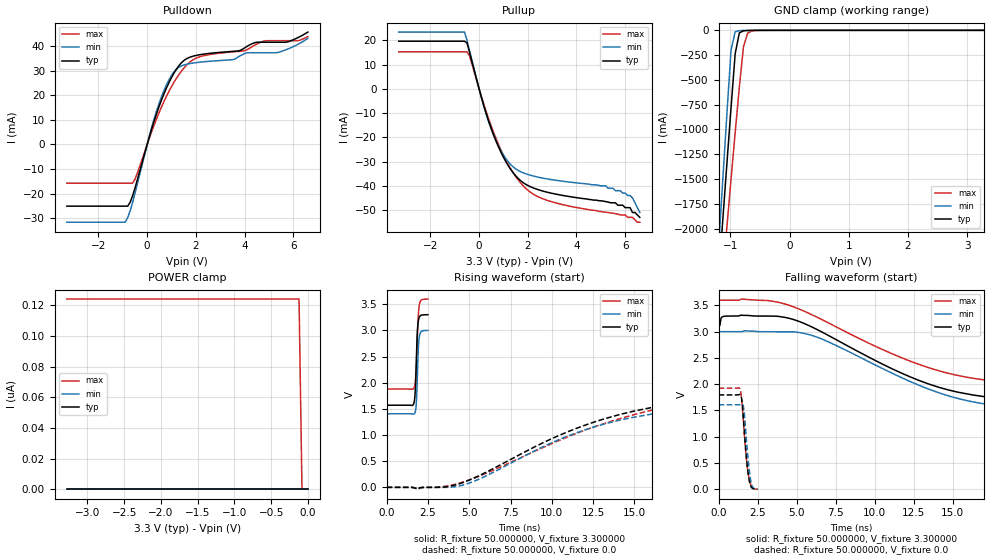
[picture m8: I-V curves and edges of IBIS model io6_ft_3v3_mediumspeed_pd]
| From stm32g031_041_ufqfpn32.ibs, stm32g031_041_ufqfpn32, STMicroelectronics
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|   Model io6_ft_3v3_mediumspeed_pd
[Model]  io6_ft_3v3_mediumspeed_pd
Model_type I/O
Polarity   Non-Inverting
Enable   Active-Low
Vinl =   0.990000V
Vinh =   2.310000V
Vmeas =  1.650000V
Cref =   50.000000pF
Rref =   100.000000M
Vref =   0.0V
C_comp   1.290400pF   1.272500pF   1.305600pF
[Temperature Range]   25.000000   -40.000000   0.125000k
[Pullup Reference]   3.300000V   3.000000V   3.600000V
[Pulldown Reference]   0.0V   0.0V   0.0V
[POWER Clamp Reference]   3.300000V   3.000000V   3.600000V
[GND Clamp Reference]   0.0V   0.0V   0.0V
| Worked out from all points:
|   slope of the pulldown table from 0 to 0.495 V, typ, clamps not added: 31.8 ohm
|   slope of the pullup table from 0 to 0.495 V, typ, clamps not added: 30.4 ohm
|   GND clamp passes 1 mA (typ) near -0.65 V on its own axis
|   rising waveform, R_fixture 50.000000, V_fixture 3.300000: 20-80 % time 114ps typ, 109ps min, 129ps max; typ from 1.57 V to 3.3 V
|   rising waveform, R_fixture 50.000000, V_fixture 0.0: 20-80 % time 8.23ns typ, 7.46ns min, 10.1ns max; typ from 0 V to 1.79 V
|   falling waveform, R_fixture 50.000000, V_fixture 3.300000: 20-80 % time 7.53ns typ, 7.46ns min, 8.06ns max; typ from 3.3 V to 1.57 V
|   falling waveform, R_fixture 50.000000, V_fixture 0.0: 20-80 % time 299ps typ, 288ps min, 331ps max; typ from 1.79 V to 0 V
[Pulldown]
|Voltage   I(typ)   I(min)   I(max)
-3.3V     -25.03mA   -31.54mA   -15.7mA
-900mV    -25.03mA   -31.54mA   -15.7mA
-700mV    -23.48mA   -26.95mA   -15.7mA
-500mV    -17.69mA   -19.75mA   -14.07mA
100mV     3.479mA    3.853mA    2.862mA
500mV     15.71mA    16.96mA    13.17mA
900mV     25.22mA    26.33mA    21.66mA
1.3V      31.91mA    31.32mA    28.29mA
2.2V      36.48mA    33.43mA    35.69mA
4.1V      39.78mA    37.21mA    38.43mA
5.4V      41.49mA    37.39mA    42.11mA
6.6V      45.6mA     43.05mA    43.74mA
[Pullup]
|Voltage   I(typ)   I(min)   I(max)
-3.3V     19.64mA    23.39mA    15.25mA
-600mV    19.64mA    23.39mA    15.25mA
-500mV    18.98mA    20.19mA    15.25mA
-400mV    15.37mA    16.06mA    13.73mA
100mV     -3.672mA   -3.825mA   -3.371mA
600mV     -19.12mA   -19.15mA   -18.08mA
1.2V      -31.74mA   -30.12mA   -31.25mA
1.8V      -38.62mA   -34.59mA   -39.86mA
3V        -43.11mA   -37.48mA   -46.63mA
5.8V      -48mA      -42mA      -52mA
6.3V      -51mA      -45mA      -53mA
6.6V      -53mA      -51mA      -55mA
[GND_clamp]
|Voltage   I(typ)   I(min)   I(max)
-3.3V     -9.61A     -9.635A    -9.699A
-1.2V     -2.493A    -2.184A    -2.958A
-1.13V    -1.917A    -1.512A    -2.469A
-1.06V    -1.345A    -845.6mA   -1.983A
-990mV    -779.8mA   -200.2mA   -1.503A
-920mV    -235.6mA   -14.2mA    -1.03A
-850mV    -26.08mA   -3.351mA   -574.2mA
-780mV    -4.512mA   -1.821mA   -166.4mA
-710mV    -1.735mA   -881.8uA   -29.46mA
-640mV    -819.4uA   -295.6uA   -6.294mA
3.28V     86.85uA    64.2uA     109.1uA
[POWER_clamp]
|Voltage   I(typ)   I(min)   I(max)
-3.28V    0A         0A         124nA
-120mV    0A         0A         124nA
-80mV     0A         0A         0A
0V        0A         0A         0A
[Ramp]
| variable   typ   min   max
dV/dt_r  1.07520/8.22726n   0.96294/7.44895n   1.14666/10.09657n
dV/dt_f  1.03122/14.35073n   0.95388/7.44449n   1.02582/8.04918n
R_load = 50.000000
[Rising Waveform]
R_fixture= 50.000000
V_fixture= 3.300000
V_fixture_min= 3.000000
V_fixture_max= 3.600000
|time   V(typ)   V(min)   V(max)
0s        1.57V      1.405V     1.878V
1.542ns   1.566V     1.403V     1.875V
1.657ns   1.62V      1.402V     1.904V
1.727ns   1.831V     1.438V     1.997V
1.792ns   2.386V     1.595V     2.294V
1.852ns   2.937V     2.054V     2.801V
1.917ns   3.182V     2.646V     3.293V
1.967ns   3.246V     2.852V     3.467V
2.052ns   3.283V     2.962V     3.562V
2.492ns   3.299V     2.999V     3.598V
[Rising Waveform]
R_fixture= 50.000000
V_fixture= 0.0
V_fixture_min= 0.0
V_fixture_max= 0.0
|time   V(typ)   V(min)   V(max)
0s        3.211nV    2.528nV    185.4nV
1.922ns   -21.16mV   -33.8mV    -31.31mV
3.604ns   10.6mV     -175.7uV   23.36mV
4.565ns   85.93mV    39.17mV    95.98mV
11.53ns   1.132V     1.047V     1.035V
14.25ns   1.403V     1.294V     1.324V
16.74ns   1.562V     1.429V     1.522V
20.18ns   1.682V     1.526V     1.705V
24.42ns   1.748V     1.575V     1.819V
39.88ns   1.794V     1.606V     1.922V
[Falling Waveform]
R_fixture= 50.000000
V_fixture= 3.300000
V_fixture_min= 3.000000
V_fixture_max= 3.600000
|time   V(typ)   V(min)   V(max)
0s        3.299V     2.999V     3.598V
80.08ps   3.118V     2.999V     3.598V
240.2ps   3.282V     2.999V     3.598V
1.441ns   3.312V     2.998V     3.616V
3.844ns   3.289V     2.997V     3.557V
5.766ns   3.117V     2.945V     3.35V
12.25ns   2.14V      2.051V     2.44V
16.34ns   1.791V     1.659V     2.11V
23.54ns   1.631V     1.469V     1.946V
39.88ns   1.57V      1.405V     1.878V
[Falling Waveform]
R_fixture= 50.000000
V_fixture= 0.0
V_fixture_min= 0.0
V_fixture_max= 0.0
|time   V(typ)   V(min)   V(max)
0s        1.794V     1.606V     1.922V
1.371ns   1.804V     1.606V     1.906V
1.436ns   1.776V     1.61V      1.813V
1.491ns   1.681V     1.617V     1.66V
1.617ns   1.226V     1.52V      1.165V
1.762ns   658.1mV    1.019V     632.4mV
1.922ns   234.2mV    471.9mV    254.4mV
2.032ns   80.05mV    210mV      108.9mV
2.142ns   22.72mV    61.87mV    36.47mV
2.492ns   3.211nV    2.528nV    185.4nV
